| IBIS file stm32wba63_a65_wlcsp88_smps_usb.ibs
[IBIS ver] 4.2
[File name] stm32wba63_a65_wlcsp88_smps_usb.ibs
[File Rev] 2.0
[Date] 17-02-2025
[Source] Data Created at STMicroelectronics
[Notes]  File originated from ELDO simulations.
[Disclaimer]  This information is for modeling purpose only and is
   not guaranted. The information is subject to change without
   notice.
[Copyright] Copyright 2025 STMicroelectronics Inc.
|   Component stm32wba63_a65_wlcsp88_smps_usb
[Component] stm32wba63_a65_wlcsp88_smps_usb
[Manufacturer] STMicroelectronics
[Package]
| variable   typ   min   max
R_pkg  0  NA  NA
L_pkg  0  NA  NA
C_pkg  0  NA  NA
[Pin]   signal_name   model_name
A4  VDDRF  nc
A6  VDDRFPA  nc
A8  VCAP  nc
A10  VSSSMPS  nc
B5  OSC_IN  nc
B7  VDD  power
B9  PA9  io8_ft_100m
B11  VDDSMPS  nc
C4  VDDANA  nc
C6  PH3-BOOT0  io8_ft_100m_v33
C8  VSS  gnd
C10  PB13  io8_ft_100m_i2c
D1  RF  nc
D5  OSC_OUT  nc
D7  PA10  io8_ft_100m
D9  PB14  io8_ft_100m_i2c
D11  VLXSMPS  nc
E2  VSSRF  nc
E4  VDDHPA  nc
E6  NRST  ioreset_v33
E8  PC3  io8_ft_100m
E10  PB12  io8_ft_100m
F1  VSSRF  nc
F3  VSSRF  nc
F5  PC6  io8_ft_100m
F7  PC5  io8_ft_100m
F9  PB11  io8_ft_100m_i2c
F11  PA8  io8_ft_100m
G2  PB15  io8_ft_100m
G4  PC8  io8_ft_100m
G6  VSS  gnd
G8  PC4  io8_ft_100m
G10  PA7  io8_ft_100m_i2c_v33
H1  PC7  io8_ft_100m
H3  PB0  io8_ft_100m
H5  VSS  gnd
H7  VSS  gnd
H9  PA6  io8_ft_100m_i2c
H11  VREFP  nc
J2  PB1  io8_ft_100m_i2c
J4  PB2  io8_ft_100m_i2c_v33
J6  VSS  gnd
J8  PC1  io8_ft_100m_i2c
J10  VSSA  nc
K1  VSS  gnd
K3  PA12  io8_ft_100m
K5  VSS  gnd
K7  VSS  gnd
K9  PC0  io8_ft_100m_i2c
K11  VDDA  nc
L2  PA11  io8_ft_100m
L4  PA13  io8_ft_100m
L6  VSS  gnd
L8  PA5  io8_ft_100m
L10  PA3  io8_ft_100m
M1  VDD  power
M3  PA14  io8_ft_100m_v33
M5  PB3  io8_ft_100m_i2c
M7  PA4  io8_ft_100m_v33
M9  PB10  io8_ft_100m_i2c
M11  VDD  power
N2  PA15  io8_ft_100m_i2c
N4  PD14  io8_ft_100m_hslv
N6  PD5  io8_ft_100m
N8  PA2  io8_ft_100m_v33
N10  PA1  io8_ft_100m
P1  VSS  gnd
P3  PE0  io8_ft_100m_hslv
P5  PB5  io8_ft_100m
P7  PD9  io8_ft_100m
P9  PA0  io8_ft_100m
P11  VSS  gnd
R2  PE1  io8_ft_100m_hslv
R4  PB4  io8_ft_100m
R6  PB8  io8_ft_100m
R8  PD8  io8_ft_100m
R10  PB9  io8_ft_100m
T1  VDD  power
T3  PE2  io8_ft_100m_hslv
T5  PB7  io8_ft_100m
T7  PC14  io_ft_tamp
T9  PD6  io8_ft_100m
T11  VDDUSB  power
U2  PE3  io8_ft_100m_hslv
U4  PB6  io8_ft_100m
U6  PC13  io8_ft_100m_v33
U8  PC15  io_ft_tamp
U10  PD7  io8_ft_100m
[Package Model]   4b0-wlcsp-88-241106
[Pin Mapping]   pulldown_ref   pullup_ref   | Comment
A4  nc  nc
A6  nc  nc
A8  nc  nc
A10  nc  nc
B5  nc  nc
B7  nc  vddio
B9  gndio  vddio
B11  nc  nc
C4  nc  nc
C6  gndio  vddio
C8  gndio  nc
C10  gndio  vddio
D1  nc  nc
D5  nc  nc
D7  gndio  vddio
D9  gndio  vddio
D11  nc  nc
E2  nc  nc
E4  nc  nc
E6  gndio  vddio
E8  gndio  vddio
E10  gndio  vddio
F1  nc  nc
F3  nc  nc
F5  gndio  vddio
F7  gndio  vddio
F9  gndio  vddio
F11  gndio  vddio
G2  gndio  vddio
G4  gndio  vddio
G6  gndio  nc
G8  gndio  vddio
G10  gndio  vddio
H1  gndio  vddio
H3  gndio  vddio
H5  gndio  nc
H7  gndio  nc
H9  gndio  vddio
H11  nc  nc
J2  gndio  vddio
J4  gndio  vddio
J6  gndio  nc
J8  gndio  vddio
J10  nc  nc
K1  gndio  nc
K3  gndio  vddio
K5  gndio  nc
K7  gndio  nc
K9  gndio  vddio
K11  nc  nc
L2  gndio  vddio
L4  gndio  vddio
L6  gndio  nc
L8  gndio  vddio
L10  gndio  vddio
M1  nc  vddio
M3  gndio  vddio
M5  gndio  vddio
M7  gndio  vddio
M9  gndio  vddio
M11  nc  vddio
N2  gndio  vddio
N4  gndio  vddio
N6  gndio  vddio
N8  gndio  vddio
N10  gndio  vddio
P1  gndio  nc
P3  gndio  vddio
P5  gndio  vddio
P7  gndio  vddio  | Depending on IO usage
| P7  gndio  vddusb  | Depending on IO usage
P9  gndio  vddio
P11  gndio  nc
R2  gndio  vddio
R4  gndio  vddio
R6  gndio  vddio
R8  gndio  vddio  | Depending on IO usage
| R8  gndio  vddusb  | Depending on IO usage
R10  gndio  vddio
T1  nc  vddio
T3  gndio  vddio
T5  gndio  vddio
T7  gndio  vddio
T9  gndio  vddio
T11  nc  vddusb
U2  gndio  vddio
U4  gndio  vddio
U6  gndio  vddio
U8  gndio  vddio
U10  gndio  vddio
|[Diff Pin]  inv_pin  vdiff  tdelay_typ  tdelay_min  tdelay_max
|T9  U10  NA  NA  NA  NA
[Model Selector] io8_ft_100m
io8_ft_100m_ls_1v2  "GPIO 100MHz - 5V tolerant - low speed - 1.2V range"
io8_ft_100m_ls_1v8  "GPIO 100MHz - 5V tolerant - low speed - 1.8V range"
io8_ft_100m_ls_3v3  "GPIO 100MHz - 5V tolerant - low speed - 3.3V range"
io8_ft_100m_ms_1v2  "GPIO 100MHz - 5V tolerant - med speed - 1.2V range"
io8_ft_100m_ms_1v8  "GPIO 100MHz - 5V tolerant - med speed - 1.8V range"
io8_ft_100m_ms_3v3  "GPIO 100MHz - 5V tolerant - med speed - 3.3V range"
io8_ft_100m_fs_1v2  "GPIO 100MHz - 5V tolerant - fast speed - 1.2V range"
io8_ft_100m_fs_1v8  "GPIO 100MHz - 5V tolerant - fast speed - 1.8V range"
io8_ft_100m_fs_3v3  "GPIO 100MHz - 5V tolerant - fast speed - 3.3V range"
io8_ft_100m_hs_1v2  "GPIO 100MHz - 5V tolerant - high speed - 1.2V range"
io8_ft_100m_hs_1v8  "GPIO 100MHz - 5V tolerant - high speed - 1.8V range"
io8_ft_100m_hs_3v3  "GPIO 100MHz - 5V tolerant - high speed - 3.3V range"
[Model Selector] io8_ft_100m_hslv
io8_ft_100m_ls_1v2  "GPIO 100MHz - 5V tolerant - low speed - 1.2V range"
io8_ft_100m_ls_1v8  "GPIO 100MHz - 5V tolerant - low speed - 1.8V range"
io8_ft_100m_ls_3v3  "GPIO 100MHz - 5V tolerant - low speed - 3.3V range"
io8_ft_100m_ms_1v2  "GPIO 100MHz - 5V tolerant - med speed - 1.2V range"
io8_ft_100m_ms_1v8  "GPIO 100MHz - 5V tolerant - med speed - 1.8V range"
io8_ft_100m_ms_3v3  "GPIO 100MHz - 5V tolerant - med speed - 3.3V range"
io8_ft_100m_fs_1v2  "GPIO 100MHz - 5V tolerant - fast speed - 1.2V range"
io8_ft_100m_fs_1v8  "GPIO 100MHz - 5V tolerant - fast speed - 1.8V range"
io8_ft_100m_fs_3v3  "GPIO 100MHz - 5V tolerant - fast speed - 3.3V range"
io8_ft_100m_hs_1v2  "GPIO 100MHz - 5V tolerant - high speed - 1.2V range"
io8_ft_100m_hs_1v8  "GPIO 100MHz - 5V tolerant - high speed - 1.8V range"
io8_ft_100m_hs_3v3  "GPIO 100MHz - 5V tolerant - high speed - 3.3V range"
io8_ft_100m_hslv_ls_1v2  "GPIO 100MHz lv opt - 5V tolerant - low speed - 1.2V range"
io8_ft_100m_hslv_ls_1v8  "GPIO 100MHz lv opt - 5V tolerant - low speed - 1.8V range"
io8_ft_100m_hslv_ls_2v5  "GPIO 100MHz lv opt - 5V tolerant - low speed - 2.5V range"
io8_ft_100m_hslv_ms_1v2  "GPIO 100MHz lv opt - 5V tolerant - med speed - 1.2V range"
io8_ft_100m_hslv_ms_1v8  "GPIO 100MHz lv opt - 5V tolerant - med speed - 1.8V range"
io8_ft_100m_hslv_ms_2v5  "GPIO 100MHz lv opt - 5V tolerant - med speed - 2.5V range"
io8_ft_100m_hslv_fs_1v2  "GPIO 100MHz lv opt - 5V tolerant - fast speed - 1.2V range"
io8_ft_100m_hslv_fs_1v8  "GPIO 100MHz lv opt - 5V tolerant - fast speed - 1.8V range"
io8_ft_100m_hslv_fs_2v5  "GPIO 100MHz lv opt - 5V tolerant - fast speed - 2.5V range"
io8_ft_100m_hslv_hs_1v2  "GPIO 100MHz lv opt - 5V tolerant - high speed - 1.2V range"
io8_ft_100m_hslv_hs_1v8  "GPIO 100MHz lv opt - 5V tolerant - high speed - 1.8V range"
io8_ft_100m_hslv_hs_2v5  "GPIO 100MHz lv opt - 5V tolerant - high speed - 2.5V range"
[Model Selector] io8_ft_100m_i2c
io8_ft_100m_ls_1v2  "GPIO 100MHz - 5V tolerant - low speed - 1.2V range"
io8_ft_100m_ls_1v8  "GPIO 100MHz - 5V tolerant - low speed - 1.8V range"
io8_ft_100m_ls_3v3  "GPIO 100MHz - 5V tolerant - low speed - 3.3V range"
io8_ft_100m_ms_1v2  "GPIO 100MHz - 5V tolerant - med speed - 1.2V range"
io8_ft_100m_ms_1v8  "GPIO 100MHz - 5V tolerant - med speed - 1.8V range"
io8_ft_100m_ms_3v3  "GPIO 100MHz - 5V tolerant - med speed - 3.3V range"
io8_ft_100m_fs_1v2  "GPIO 100MHz - 5V tolerant - fast speed - 1.2V range"
io8_ft_100m_fs_1v8  "GPIO 100MHz - 5V tolerant - fast speed - 1.8V range"
io8_ft_100m_fs_3v3  "GPIO 100MHz - 5V tolerant - fast speed - 3.3V range"
io8_ft_100m_hs_1v2  "GPIO 100MHz - 5V tolerant - high speed - 1.2V range"
io8_ft_100m_hs_1v8  "GPIO 100MHz - 5V tolerant - high speed - 1.8V range"
io8_ft_100m_hs_3v3  "GPIO 100MHz - 5V tolerant - high speed - 3.3V range"
io8_ft_100m_i2c_ls_1v2  "GPIO 100MHz with I2C open-drain - 5V tolerant - low speed - 1.2V range"
io8_ft_100m_i2c_ls_1v8  "GPIO 100MHz with I2C open-drain - 5V tolerant - low speed - 1.8V range"
io8_ft_100m_i2c_ls_3v3  "GPIO 100MHz with I2C open-drain - 5V tolerant - low speed - 3.3V range"
io8_ft_100m_i2c_ms_1v2  "GPIO 100MHz with I2C open-drain - 5V tolerant - med speed - 1.2V range"
io8_ft_100m_i2c_ms_1v8  "GPIO 100MHz with I2C open-drain - 5V tolerant - med speed - 1.8V range"
io8_ft_100m_i2c_ms_3v3  "GPIO 100MHz with I2C open-drain - 5V tolerant - med speed - 3.3V range"
io8_ft_100m_i2c_fs_1v2  "GPIO 100MHz with I2C open-drain - 5V tolerant - fast speed - 1.2V range"
io8_ft_100m_i2c_fs_1v8  "GPIO 100MHz with I2C open-drain - 5V tolerant - fast speed - 1.8V range"
io8_ft_100m_i2c_fs_3v3  "GPIO 100MHz with I2C open-drain - 5V tolerant - fast speed - 3.3V range"
io8_ft_100m_i2c_hs_1v2  "GPIO 100MHz with I2C open-drain - 5V tolerant - high speed - 1.2V range"
io8_ft_100m_i2c_hs_1v8  "GPIO 100MHz with I2C open-drain - 5V tolerant - high speed - 1.8V range"
io8_ft_100m_i2c_hs_3v3  "GPIO 100MHz with I2C open-drain - 5V tolerant - high speed - 3.3V range"
io8_ft_100m_i2c_fmp_3v3  "GPIO 100MHz with I2C fm+ open-drain - 5V tolerant - low speed - 3.3V range"
io8_ft_100m_i2c_fmp_1v8  "GPIO 100MHz with I2C fm+ open-drain - 5V tolerant - low speed - 1.8V range"
io8_ft_100m_i2c_fmp_1v2  "GPIO 100MHz with I2C fm+ open-drain - 5V tolerant - low speed - 1.2V range"
[Model Selector] io8_ft_100m_i2c_v33
io8_ft_100m_v33_ls_1v2  "GPIO_V33 100MHz - 5V tolerant - low speed - 1.2V range"
io8_ft_100m_v33_ls_1v8  "GPIO_V33 100MHz - 5V tolerant - low speed - 1.8V range"
io8_ft_100m_v33_ls_3v3  "GPIO_V33 100MHz - 5V tolerant - low speed - 3.3V range"
io8_ft_100m_v33_ms_1v2  "GPIO_V33 100MHz - 5V tolerant - med speed - 1.2V range"
io8_ft_100m_v33_ms_1v8  "GPIO_V33 100MHz - 5V tolerant - med speed - 1.8V range"
io8_ft_100m_v33_ms_3v3  "GPIO_V33 100MHz - 5V tolerant - med speed - 3.3V range"
io8_ft_100m_v33_fs_1v2  "GPIO_V33 100MHz - 5V tolerant - fast speed - 1.2V range"
io8_ft_100m_v33_fs_1v8  "GPIO_V33 100MHz - 5V tolerant - fast speed - 1.8V range"
io8_ft_100m_v33_fs_3v3  "GPIO_V33 100MHz - 5V tolerant - fast speed - 3.3V range"
io8_ft_100m_v33_hs_1v2  "GPIO_V33 100MHz - 5V tolerant - high speed - 1.2V range"
io8_ft_100m_v33_hs_1v8  "GPIO_V33 100MHz - 5V tolerant - high speed - 1.8V range"
io8_ft_100m_v33_hs_3v3  "GPIO_V33 100MHz - 5V tolerant - high speed - 3.3V range"
io8_ft_100m_i2c_v33_ls_1v2  "GPIO_V33 100MHz with I2C open-drain - 5V tolerant - low speed - 1.2V range"
io8_ft_100m_i2c_v33_ls_1v8  "GPIO_V33 100MHz with I2C open-drain - 5V tolerant - low speed - 1.8V range"
io8_ft_100m_i2c_v33_ls_3v3  "GPIO_V33 100MHz with I2C open-drain - 5V tolerant - low speed - 3.3V range"
io8_ft_100m_i2c_v33_ms_1v2  "GPIO_V33 100MHz with I2C open-drain - 5V tolerant - med speed - 1.2V range"
io8_ft_100m_i2c_v33_ms_1v8  "GPIO_V33 100MHz with I2C open-drain - 5V tolerant - med speed - 1.8V range"
io8_ft_100m_i2c_v33_ms_3v3  "GPIO_V33 100MHz with I2C open-drain - 5V tolerant - med speed - 3.3V range"
io8_ft_100m_i2c_v33_fs_1v2  "GPIO_V33 100MHz with I2C open-drain - 5V tolerant - fast speed - 1.2V range"
io8_ft_100m_i2c_v33_fs_1v8  "GPIO_V33 100MHz with I2C open-drain - 5V tolerant - fast speed - 1.8V range"
io8_ft_100m_i2c_v33_fs_3v3  "GPIO_V33 100MHz with I2C open-drain - 5V tolerant - fast speed - 3.3V range"
io8_ft_100m_i2c_v33_hs_1v2  "GPIO_V33 100MHz with I2C open-drain - 5V tolerant - high speed - 1.2V range"
io8_ft_100m_i2c_v33_hs_1v8  "GPIO_V33 100MHz with I2C open-drain - 5V tolerant - high speed - 1.8V range"
io8_ft_100m_i2c_v33_hs_3v3  "GPIO_V33 100MHz with I2C open-drain - 5V tolerant - high speed - 3.3V range"
io8_ft_100m_i2c_fmp_v33_1v2  "GPIO_V33 100MHz with I2C fm+ open-drain - 5V tolerant - low speed - 1.2V range"
io8_ft_100m_i2c_fmp_v33_1v8  "GPIO_V33 100MHz with I2C fm+ open-drain - 5V tolerant - low speed - 1.8V range"
io8_ft_100m_i2c_fmp_v33_3v3  "GPIO_V33 100MHz with I2C fm+ open-drain - 5V tolerant - low speed - 3.3V range"
[Model Selector] io8_ft_100m_v33
io8_ft_100m_v33_ls_1v2  "GPIO_V33 100MHz - 5V tolerant - low speed - 1.2V range"
io8_ft_100m_v33_ls_1v8  "GPIO_V33 100MHz - 5V tolerant - low speed - 1.8V range"
io8_ft_100m_v33_ls_3v3  "GPIO_V33 100MHz - 5V tolerant - low speed - 3.3V range"
io8_ft_100m_v33_ms_1v2  "GPIO_V33 100MHz - 5V tolerant - med speed - 1.2V range"
io8_ft_100m_v33_ms_1v8  "GPIO_V33 100MHz - 5V tolerant - med speed - 1.8V range"
io8_ft_100m_v33_ms_3v3  "GPIO_V33 100MHz - 5V tolerant - med speed - 3.3V range"
io8_ft_100m_v33_fs_1v2  "GPIO_V33 100MHz - 5V tolerant - fast speed - 1.2V range"
io8_ft_100m_v33_fs_1v8  "GPIO_V33 100MHz - 5V tolerant - fast speed - 1.8V range"
io8_ft_100m_v33_fs_3v3  "GPIO_V33 100MHz - 5V tolerant - fast speed - 3.3V range"
io8_ft_100m_v33_hs_1v2  "GPIO_V33 100MHz - 5V tolerant - high speed - 1.2V range"
io8_ft_100m_v33_hs_1v8  "GPIO_V33 100MHz - 5V tolerant - high speed - 1.8V range"
io8_ft_100m_v33_hs_3v3  "GPIO_V33 100MHz - 5V tolerant - high speed - 3.3V range"
[Model Selector] io_ft_tamp
io_ft_tamp_ls_1v2 "io8_ft tamp low speed @ 1.2V"
io_ft_tamp_ls_1v8 "io8_ft tamp low speed @ 1.8V"
io_ft_tamp_ls_3v3 "io8_ft tamp low speed @ 3.3V"
io_ft_tamp_ms_1v2 "io8_ft tamp med speed @ 1.2V"
io_ft_tamp_ms_1v8 "io8_ft tamp med speed @ 1.8V"
io_ft_tamp_ms_3v3 "io8_ft tamp med speed @ 3.3V"
io_ft_tamp_fs_1v2 "io8_ft tamp fast speed @ 1.2V"
io_ft_tamp_fs_1v8 "io8_ft tamp fast speed @ 1.8V"
io_ft_tamp_fs_3v3 "io8_ft tamp fast speed @ 3.3V"
io_ft_tamp_hs_1v2 "io8_ft tamp high speed @ 1.2V"
io_ft_tamp_hs_1v8 "io8_ft tamp high speed @ 1.8V"
io_ft_tamp_hs_3v3 "io8_ft tamp high speed @ 3.3V"
[Model Selector] ioreset_v33
ioreset_v33_1v2 "Reset PAD. 5V tolerant. 1.2V range"
ioreset_v33_1v8 "Reset PAD. 5V tolerant. 1.8V range"
ioreset_v33_3v3 "Reset PAD. 5V tolerant. 3.3V range"
[Define Package Model]  4b0-wlcsp-88-241106
[Manufacturer]  Unknown
[OEM]  Unknown
[Description]  None
[Number Of Pins]  73
[Pin Numbers]
| Pin Num   Terminal Name
D1 | RF
E6 | NRST
B5 | OSC_IN
D5 | OSC_OUT
P9 | PA0
N10 | PA1
N8 | PA2
L10 | PA3
M7 | PA4
L8 | PA5
H9 | PA6
G10 | PA7
F11 | PA8
B9 | PA9
D7 | PA10
L2 | PA11
K3 | PA12
L4 | PA13
M3 | PA14
N2 | PA15
H3 | PB0
J2 | PB1
J4 | PB2
M5 | PB3
R4 | PB4
P5 | PB5
U4 | PB6
T5 | PB7
R6 | PB8
R10 | PB9
M9 | PB10
F9 | PB11
E10 | PB12
C10 | PB13
D9 | PB14
G2 | PB15
K9 | PC0
J8 | PC1
E8 | PC3
G8 | PC4
F7 | PC5
F5 | PC6
H1 | PC7
G4 | PC8
U6 | PC13
T7 | PC14
U8 | PC15
N6 | PD5
T9 | PD6
U10 | PD7
R8 | PD8
P7 | PD9
N4 | PD14
P3 | PE0
R2 | PE1
T3 | PE2
U2 | PE3
C6 | PH3-BOOT0
B7 | VDD
A8 | VCAP
K11 | VDDA
C4 | VDDANA
E4 | VDDHPA
A4 | VDDRF
A6 | VDDRFPA
B11 | VDDSMPS
T11 | VDDUSB
D11 | VLXSMPS
H11 | VREFP
C8 | VSS
J10 | VSSA
E2 | VSSRF
A10 | VSSSMPS
|[Merged Pins]  B7
|M1  |  VDD
|M11  |  VDD
|T1  |  VDD
|[Merged Pins]  C8
|G6  |  VSS
|H5  |  VSS
|H7  |  VSS
|J6  |  VSS
|K1  |  VSS
|K5  |  VSS
|K7  |  VSS
|L6  |  VSS
|P1  |  VSS
|P11  |  VSS
|[Merged Pins]  E2
|F1  |  VSSRF
|F3  |  VSSRF
[Model Data]
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[End Model Data]
[End Package Model]
|End [Component]
| Models and submodels in the file (81): io8_ft_100m_fs_1v2 (I/O), io8_ft_100m_fs_1v8 (I/O), io8_ft_100m_fs_3v3 (I/O), io8_ft_100m_hs_1v2 (I/O), io8_ft_100m_hs_1v8 (I/O), io8_ft_100m_hs_3v3 (I/O), io8_ft_100m_hslv_fs_1v2 (I/O), io8_ft_100m_hslv_fs_1v8 (I/O), io8_ft_100m_hslv_fs_2v5 (I/O), io8_ft_100m_hslv_hs_1v2 (I/O), io8_ft_100m_hslv_hs_1v8 (I/O), io8_ft_100m_hslv_hs_2v5 (I/O), io8_ft_100m_hslv_ls_1v2 (I/O), io8_ft_100m_hslv_ls_1v8 (I/O), io8_ft_100m_hslv_ls_2v5 (I/O), io8_ft_100m_hslv_ms_1v2 (I/O), io8_ft_100m_hslv_ms_1v8 (I/O), io8_ft_100m_hslv_ms_2v5 (I/O), io8_ft_100m_i2c_fmp_1v2 (I/O_open_drain), io8_ft_100m_i2c_fmp_1v8 (I/O_open_drain), io8_ft_100m_i2c_fmp_3v3 (I/O_open_drain), io8_ft_100m_i2c_fmp_v33_1v2 (I/O_open_drain), io8_ft_100m_i2c_fmp_v33_1v8 (I/O_open_drain), io8_ft_100m_i2c_fmp_v33_3v3 (I/O_open_drain), io8_ft_100m_i2c_fs_1v2 (I/O_open_drain), io8_ft_100m_i2c_fs_1v8 (I/O_open_drain), io8_ft_100m_i2c_fs_3v3 (I/O_open_drain), io8_ft_100m_i2c_hs_1v2 (I/O_open_drain), io8_ft_100m_i2c_hs_1v8 (I/O_open_drain), io8_ft_100m_i2c_hs_3v3 (I/O_open_drain), io8_ft_100m_i2c_ls_1v2 (I/O_open_drain), io8_ft_100m_i2c_ls_1v8 (I/O_open_drain), io8_ft_100m_i2c_ls_3v3 (I/O_open_drain), io8_ft_100m_i2c_ms_1v2 (I/O_open_drain), io8_ft_100m_i2c_ms_1v8 (I/O_open_drain), io8_ft_100m_i2c_ms_3v3 (I/O_open_drain), io8_ft_100m_i2c_v33_fs_1v2 (I/O_open_drain), io8_ft_100m_i2c_v33_fs_1v8 (I/O_open_drain), io8_ft_100m_i2c_v33_fs_3v3 (I/O_open_drain), io8_ft_100m_i2c_v33_hs_1v2 (I/O_open_drain), io8_ft_100m_i2c_v33_hs_1v8 (I/O_open_drain), io8_ft_100m_i2c_v33_hs_3v3 (I/O_open_drain), io8_ft_100m_i2c_v33_ls_1v2 (I/O_open_drain), io8_ft_100m_i2c_v33_ls_1v8 (I/O_open_drain), io8_ft_100m_i2c_v33_ls_3v3 (I/O_open_drain), io8_ft_100m_i2c_v33_ms_1v2 (I/O_open_drain), io8_ft_100m_i2c_v33_ms_1v8 (I/O_open_drain), io8_ft_100m_i2c_v33_ms_3v3 (I/O_open_drain), io8_ft_100m_ls_1v2 (I/O), io8_ft_100m_ls_1v8 (I/O), io8_ft_100m_ls_3v3 (I/O), io8_ft_100m_ms_1v2 (I/O), io8_ft_100m_ms_1v8 (I/O), io8_ft_100m_ms_3v3 (I/O), io8_ft_100m_v33_fs_1v2 (I/O), io8_ft_100m_v33_fs_1v8 (I/O), io8_ft_100m_v33_fs_3v3 (I/O), io8_ft_100m_v33_hs_1v2 (I/O), io8_ft_100m_v33_hs_1v8 (I/O), io8_ft_100m_v33_hs_3v3 (I/O), io8_ft_100m_v33_ls_1v2 (I/O), io8_ft_100m_v33_ls_1v8 (I/O), io8_ft_100m_v33_ls_3v3 (I/O), io8_ft_100m_v33_ms_1v2 (I/O), io8_ft_100m_v33_ms_1v8 (I/O), io8_ft_100m_v33_ms_3v3 (I/O), io_ft_tamp_fs_1v2 (I/O), io_ft_tamp_fs_1v8 (I/O), io_ft_tamp_fs_3v3 (I/O), io_ft_tamp_hs_1v2 (I/O), io_ft_tamp_hs_1v8 (I/O), io_ft_tamp_hs_3v3 (I/O), io_ft_tamp_ls_1v2 (I/O), io_ft_tamp_ls_1v8 (I/O), io_ft_tamp_ls_3v3 (I/O), io_ft_tamp_ms_1v2 (I/O), io_ft_tamp_ms_1v8 (I/O), io_ft_tamp_ms_3v3 (I/O), ioreset_v33_1v2 (I/O_open_drain), ioreset_v33_1v8 (I/O_open_drain)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
